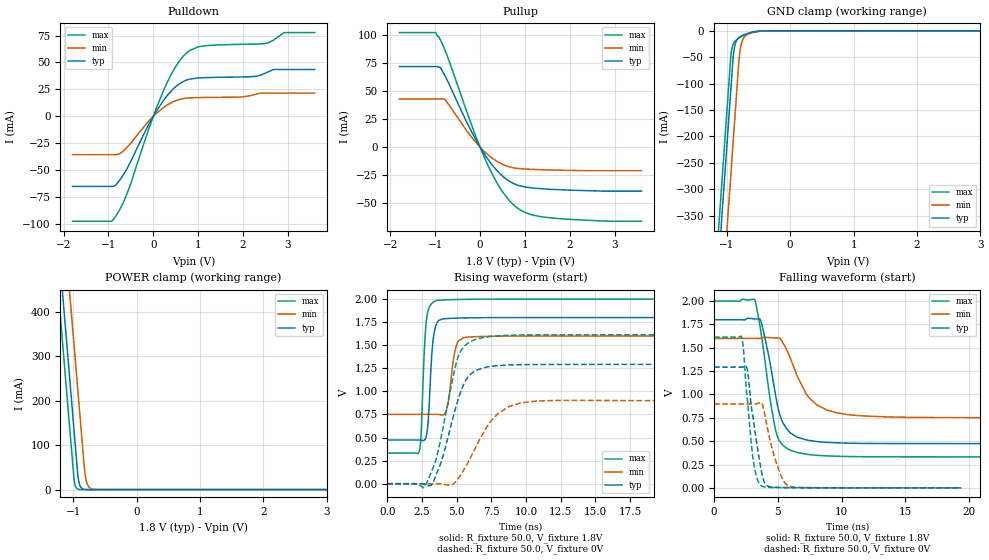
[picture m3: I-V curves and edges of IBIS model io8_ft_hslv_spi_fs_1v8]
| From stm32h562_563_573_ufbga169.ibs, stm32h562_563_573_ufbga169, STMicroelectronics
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[Model]   io8_ft_hslv_spi_fs_1v8
Model_type I/O
Polarity   Non-Inverting
Enable   Active-Low
| CAP_THRESHOLD on pad IOFT is "UDTCAPC" :
| Rising=20.0% of vddiom   Falling=80.0% of vddiom
| C_comp min and max val. don't necessarily correlate with the min and max pvt
| but are the smallest and greatest pad capacitance found.
| var   typ   min   max
C_comp   4.56172pF  4.45455pF  4.74994pF
|C_comp_pullup   2.85885pF  2.67925pF  2.77985pF
|C_comp_pulldown   1.70287pF  1.77530pF  1.97009pF
Vinl = 480.0mV
Vinh = 1.4V
Vmeas = 900.0mV   | Reference voltage for timing measurements
Cref  = 50.0pF   | Timing specification test load capacitance value
Rref  = 100.0MOhm   | Timing specification test load resistance value
Vref  = 900.0mV   | Timing specification test load voltage
[Model Spec]
| TIME_THRESHOLD on pin ZIV11 is "CMOS" :
| Rising=40.0% of vdd   Falling=60.0% of vdd
Vinl 703.80000mV 631.80000mV 784.80000mV
Vinh 1.06220V 937.20000mV 1.16620V
| variable   typ   min   max
[Temperature Range] 25.0 125.0 -40.0
| variable   typ   min   max
[Voltage Range] 1.8V 1.6V 2.0V
| variable   typ   min   max
[POWER Clamp Reference] 1.8V 1.6V 2.0V
| variable   typ   min   max
[GND Clamp Reference] 0V 0V 0V
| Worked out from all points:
|   slope of the pulldown table from 0 to 0.27 V, typ, clamps not added: 15.8 ohm
|   slope of the pullup table from 0 to 0.27 V, typ, clamps not added: 17.1 ohm
|   GND clamp passes 1 mA (typ) near -0.52 V on its own axis
|   POWER clamp passes 1 mA (typ) near -0.84 V on its own axis
|   rising waveform, R_fixture 50.0, V_fixture 1.8V: 20-80 % time 313ps typ, 435ps min, 285ps max; typ from 0.474 V to 1.8 V
|   falling waveform, R_fixture 50.0, V_fixture 1.8V: 20-80 % time 1.16ns typ, 1.94ns min, 1.08ns max; typ from 1.8 V to 0.474 V
|   rising waveform, R_fixture 50.0, V_fixture 0V: 20-80 % time 1.46ns typ, 2.08ns min, 1.33ns max; typ from 0 V to 1.29 V
|   falling waveform, R_fixture 50.0, V_fixture 0V: 20-80 % time 810ps typ, 1.04ns min, 638ps max; typ from 1.29 V to 0 V
[POWER Clamp]
-1.8V     1.518A     1.709A     1.407A
-1.23V    548.8mA    740.2mA    437.5mA
-1.16V    429.8mA    621.2mA    318.5mA
-1.05V    242.8mA    434.2mA    131.5mA
-980mV    123.8mA    315.2mA    17.95mA
-930mV    38.81mA    230.2mA    1.49mA
-910mV    17.82mA    196.2mA    550.8uA
-890mV    8.18mA     162.2mA    203.5uA
-810mV    363.5uA    33.6mA     3.797uA
-770mV    76.62uA    10.47mA    518.8nA
-710mV    7.417uA    1.822mA    26.38nA
3.6V      0A         0A         0A
[GND Clamp]
-1.8V     -1.581A    -1.742A    -1.516A
-1.24V    -628.8mA   -789.9mA   -564.1mA
-1.05V    -305.8mA   -466.9mA   -241.1mA
-940mV    -118.8mA   -279.9mA   -54.1mA
-930mV    -101.8mA   -262.9mA   -41.86mA
-900mV    -51.51mA   -211.9mA   -25.34mA
-880mV    -32.22mA   -177.9mA   -21mA
-810mV    -13.02mA   -59.5mA    -13.82mA
-770mV    -9.8mA     -24.99mA   -11mA
-680mV    -5.275mA   -7.288mA   -5.917mA
-400mV    -107uA     -349.1uA   -42.51uA
3.6V      5.392nA    968.2nA    261.3pA
| variable   typ   min   max
[Pullup Reference] 1.8V 1.6V 2.0V
| variable   typ   min   max
[Pulldown Reference] 0V 0V 0V
[Pullup]
-1.8V     71.54mA    42.73mA    101.8mA
-990mV    71.54mA    42.73mA    101.8mA
-920mV    70.86mA    42.73mA    98.07mA
-880mV    70.36mA    42.73mA    94.9mA
-790mV    63.86mA    42.48mA    86.8mA
-310mV    23.12mA    15.21mA    32.96mA
150mV     -9.305mA   -5.807mA   -13.91mA
500mV     -25.61mA   -15.24mA   -39.45mA
830mV     -33.6mA    -18.8mA    -53.95mA
1.18V     -36.29mA   -19.75mA   -60.37mA
1.56V     -37.38mA   -20.24mA   -62.7mA
3.6V      -38.97mA   -20.89mA   -65.81mA
[Pulldown]
-1.8V     -65.02mA   -35.56mA   -97.42mA
-940mV    -65.02mA   -35.56mA   -97.42mA
-850mV    -64.17mA   -35.56mA   -93.5mA
-570mV    -47.32mA   -28.01mA   -70.04mA
-120mV    -9.088mA   -5.279mA   -14.07mA
250mV     16.04mA    8.832mA    26.05mA
550mV     29.17mA    15.25mA    49.41mA
780mV     34.17mA    17.07mA    60.14mA
1.18V     35.97mA    17.56mA    65.65mA
2.49V     39.87mA    21.59mA    67.54mA
2.92V     43.47mA    21.59mA    77.77mA
3.6V      43.47mA    21.59mA    77.77mA
[Ramp]
dV/dt_r 775.79828mV/1.45705ns 538.9699mV/2.07082ns 968.315mV/1.32956ns
dV/dt_f 795.78696mV/1.16219ns 508.9792mV/1.89712ns 1.00099V/1.07865ns
R_load = 50.0
| Removed startup time: 0s 0s 0s  .
| Removed end time: 19.4ns.
[Rising Waveform]
R_fixture   = 50.0
V_fixture   = 1.8V
V_fixture_min = 1.6V
V_fixture_max = 2.0V
0s        473.7mV    751.7mV    331.7mV
2.3ns     473.9mV    751.7mV    348mV
2.45ns    471.7mV    751.7mV    568.8mV
2.65ns    469.2mV    751.8mV    1.372V
2.8ns     508mV      751.8mV    1.738V
3.4ns     1.651V     752.2mV    1.976V
4.25ns    1.788V     791.3mV    1.992V
4.9ns     1.794V     1.451V     1.996V
5.55ns    1.797V     1.585V     1.997V
19.4ns    1.8V       1.6V       2V
| Removed startup time: 0s 0s 0s  .
| Removed end time: 39.4ns.
[Falling Waveform]
R_fixture   = 50.0
V_fixture   = 1.8V
V_fixture_min = 1.6V
V_fixture_max = 2.0V
0s        1.8V       1.6V       2V
3.2ns     1.808V     1.6V       2.013V
3.75ns    1.748V     1.606V     1.601V
4.4ns     1.331V     1.609V     948.9mV
4.9ns     936.5mV    1.604V     582.2mV
5.4ns     697.2mV    1.554V     456.1mV
6.45ns    547.1mV    1.223V     381.4mV
8.05ns    496mV      890mV      348.6mV
10.45ns   478.6mV    785.1mV    335.8mV
39.4ns    473.7mV    751.7mV    331.7mV
| Removed startup time: 0s 0s 0s  .
| Removed end time: 39.3ns.
[Rising Waveform]
R_fixture   = 50.0
V_fixture   = 0V
V_fixture_min = 0V
V_fixture_max = 0V
0s        134.7nV    547.1nV    93.85nV
2.7ns     -10.04mV   -7.453uV   -30.33mV
3.2ns     -13.19mV   -31.56uV   135.3mV
3.8ns     198.3mV    -114.4uV   444.7mV
5.1ns     907.5mV    54.53mV    1.372V
5.7ns     1.13V      198.1mV    1.51V
6.5ns     1.233V     433.7mV    1.57V
8ns       1.28V      762.3mV    1.603V
10.5ns    1.291V     892.2mV    1.613V
39.3ns    1.293V     898.3mV    1.614V
| Removed startup time: 0s 0s 0s  .
| Removed end time: 19.4ns.
[Falling Waveform]
R_fixture   = 50.0
V_fixture   = 0V
V_fixture_min = 0V
V_fixture_max = 0V
0s        1.293V     898.3mV    1.614V
2.15ns    1.293V     898.3mV    1.62V
2.3ns     1.295V     898.3mV    1.492V
2.6ns     1.271V     898.3mV    960mV
3.05ns    763.1mV    898.2mV    316.7mV
3.75ns    155.1mV    905.3mV    18.19mV
4.1ns     29.11mV    696.9mV    7.038mV
5ns       4.718mV    222.4mV    3.1mV
5.95ns    2.496mV    15.53mV    1.849mV
19.4ns    10.63uV    67.1uV     1.746uV
